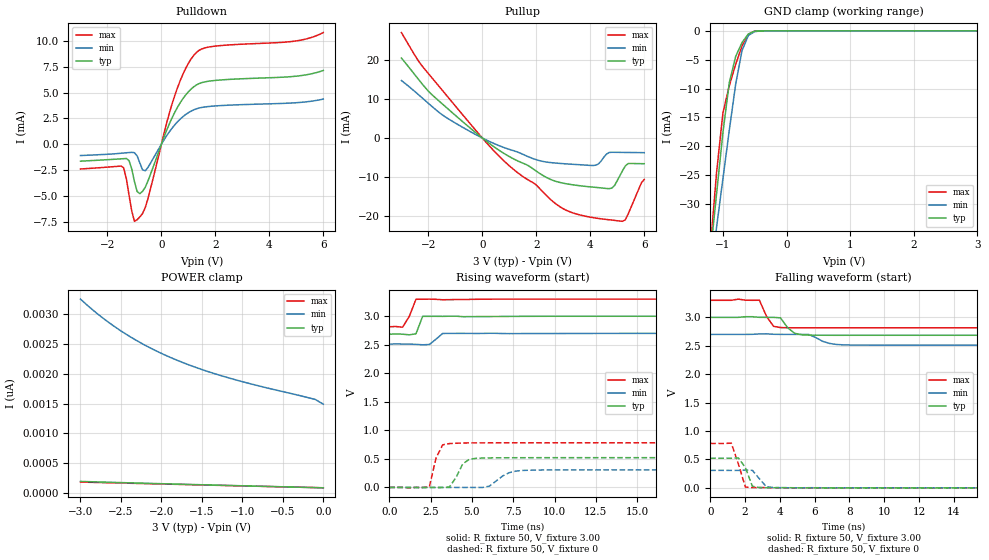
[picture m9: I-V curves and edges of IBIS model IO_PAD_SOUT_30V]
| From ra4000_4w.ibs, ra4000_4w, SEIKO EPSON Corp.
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[Model]   IO_PAD_SOUT_30V
Model_type 3-state
Enable Active-High
Polarity Non-Inverting
Vmeas=1.50
C_comp   2.5p   2.0p   3.0p
[Temperature Range] 25   125   -40
[Voltage Range]   3.00   2.70   3.30
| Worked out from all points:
|   slope of the pulldown table from 0 to 0.45 V, typ, clamps not added: 158 ohm
|   slope of the pullup table from 0 to 0.45 V, typ, clamps not added: 193 ohm
|   GND clamp passes 1 mA (typ) near -0.63 V on its own axis
|   falling waveform, R_fixture 50, V_fixture 3.00: 20-80 % time 567ps typ, 847ps min, 507ps max; typ from 3 V to 2.69 V
|   falling waveform, R_fixture 50, V_fixture 0: 20-80 % time 451ps typ, 516ps min, 488ps max; typ from 0.521 V to 0 V
|   rising waveform, R_fixture 50, V_fixture 3.00: 20-80 % time 249ps typ, 471ps min, 458ps max; typ from 2.69 V to 3 V
|   rising waveform, R_fixture 50, V_fixture 0: 20-80 % time 597ps typ, 943ps min, 481ps max; typ from 0 V to 0.521 V
[Pullup]
-3V       20.45mA    14.69mA    26.95mA
-2.4V     15.29mA    11.28mA    20.02mA
-1.9V     11.29mA    8.266mA    15.65mA
300mV     -1.589mA   -1mA       -2.327mA
1.2V      -5.477mA   -3.33mA    -8.267mA
2V        -8.47mA    -5.542mA   -12.03mA
2.9V      -11.4mA    -6.501mA   -17.67mA
4.2V      -12.61mA   -6.947mA   -20.45mA
4.8V      -12.81mA   -3.639mA   -20.96mA
5.2V      -8.293mA   -3.674mA   -21.28mA
5.4V      -6.536mA   -3.691mA   -19.5mA
6V        -6.57mA    -3.743mA   -10.6mA
[Pulldown]
-3V       -1.645mA   -1.099mA   -2.404mA
-1.4V     -1.401mA   -852.5uA   -2.281mA
-1.2V     -1.594mA   -809uA     -4.933mA
-1V       -3.61mA    -823.9uA   -7.472mA
-800mV    -4.793mA   -1.813mA   -7.046mA
-600mV    -4.172mA   -2.579mA   -6.158mA
500mV     3.112mA    1.89mA     4.757mA
900mV     4.773mA    2.879mA    7.349mA
1.3V      5.744mA    3.433mA    8.902mA
2V        6.182mA    3.71mA     9.508mA
5V        6.596mA    4.022mA    10.01mA
6V        7.149mA    4.375mA    10.82mA
[GND Clamp]
-3V       -252.2mA   -212.5mA   -302.7mA
-1.2V     -38.93mA   -42.42mA   -37.92mA
-1.1V     -28.21mA   -33.99mA   -24.54mA
-1V       -17.61mA   -25.59mA   -14.21mA
-900mV    -8.987mA   -17.22mA   -9.509mA
-800mV    -4.449mA   -9.275mA   -5.815mA
-700mV    -2.032mA   -3.425mA   -2.638mA
-600mV    -545.3uA   -804.5uA   -605.9uA
-500mV    -56.89uA   -135.5uA   -35.53uA
-400mV    -3.147uA   -16.88uA   -734nA
3V        91.06pA    1.636nA    82.41pA
[POWER Clamp]
-3V       198.6pA    3.245nA    187.7pA
-2.8V     190.6pA    3.01nA     181.3pA
-2.7V     186.7pA    2.904nA    178.1pA
-2.5V     179pA      2.713nA    171.7pA
-2.4V     175.2pA    2.627nA    168.5pA
-2.2V     167.8pA    2.472nA    162.1pA
-1.9V     156.9pA    2.277nA    152.5pA
-1.6V     146.2pA    2.116nA    142.9pA
-1.3V     135.8pA    1.981nA    133.4pA
-900mV    122.1pA    1.83nA     120.7pA
-100mV    94.97pA    1.569nA    95.68pA
0V        91.06pA    1.489nA    92.43pA
[Falling Waveform]
R_fixture=50
V_fixture=3.00
V_fixture_min=2.70
V_fixture_max=3.30
0s        3V         2.7V       3.3V
2.828ns   3V         2.708V     3.301V
3.232ns   3V         2.71V      3.021V
3.636ns   3V         2.702V     2.843V
4.04ns    2.991V     2.7V       2.82V
4.848ns   2.72V      2.7V       2.816V
5.657ns   2.687V     2.7V       2.816V
6.869ns   2.685V     2.54V      2.817V
8.081ns   2.685V     2.513V     2.817V
40ns      2.685V     2.511V     2.817V
[Falling Waveform]
R_fixture=50
V_fixture=0
V_fixture_min=0
V_fixture_max=0
0s        521.3mV    307.8mV    782mV
1.212ns   520.7mV    307.2mV    786.6mV
1.616ns   527.2mV    307mV      424.6mV
2.02ns    358.9mV    312.3mV    14.08mV
2.424ns   28.01mV    308.5mV    4.644mV
2.828ns   5.187mV    159.3mV    5.09mV
3.232ns   2.582mV    18.62mV    4.896mV
3.636ns   2.027mV    6.38mV     1.744mV
4.04ns    4.483mV    2.817mV    1.086mV
40ns      8.033uV    11.5uV     5.688uV
[Rising Waveform]
R_fixture=50
V_fixture=3.00
V_fixture_min=2.70
V_fixture_max=3.30
0s        2.685V     2.511V     2.816V
404ps     2.69V      2.516V     2.819V
808.1ps   2.685V     2.513V     2.809V
1.212ns   2.674V     2.511V     2.998V
1.616ns   2.692V     2.507V     3.298V
2.02ns    2.999V     2.5V       3.298V
2.424ns   2.999V     2.504V     3.3V
3.232ns   2.998V     2.699V     3.289V
6.869ns   2.996V     2.697V     3.3V
40ns      3V         2.7V       3.3V
[Rising Waveform]
R_fixture=50
V_fixture=0
V_fixture_min=0
V_fixture_max=0
0s        915.1pV    3.751nV    846.3pV
2.424ns   70.37uV    -410uV     9.915mV
2.828ns   9.171uV    -3.606mV   513.7mV
3.232ns   -1.247mV   -1.479mV   746.1mV
3.636ns   5.853mV    29.32uV    768.2mV
4.444ns   412mV      -12.01uV   778.1mV
5.253ns   510mV      -1.2mV     780.8mV
7.273ns   520.1mV    259.5mV    781.7mV
8.485ns   520.8mV    301.9mV    781.8mV
40ns      521.3mV    307.8mV    782mV
[Ramp]
R_load=50
dV/dt_r   3.128E-1/5.123E-10   1.847E-1/8.950E-10   4.692E-1/3.138E-10
dV/dt_f   1.891E-1/4.743E-10   1.135E-1/7.792E-10   2.901E-1/3.254E-10
|[End   IO_PAD_SOUT_30V
